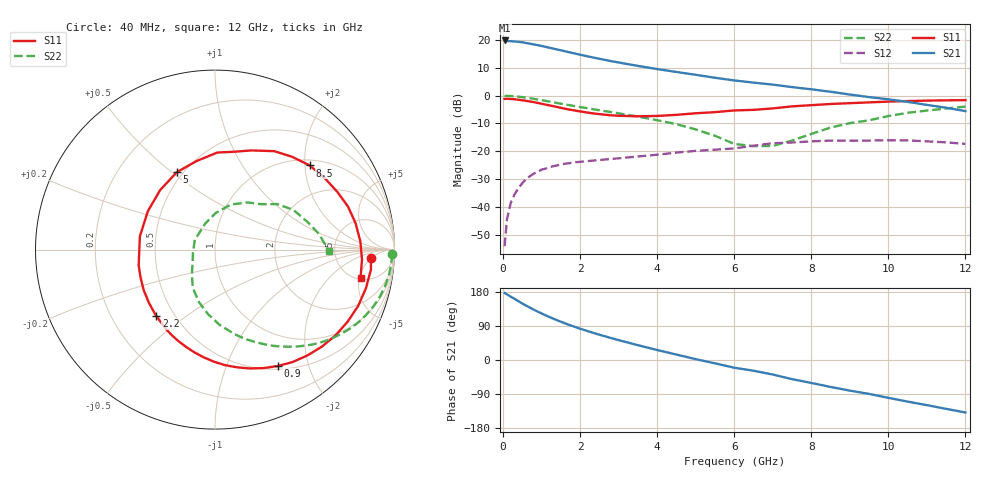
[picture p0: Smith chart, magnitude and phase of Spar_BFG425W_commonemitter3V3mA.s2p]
! Filename: 33bfg425.001
! BFG425W Field C1
! V1=8.136E-001V,V2=3.000E+000V, I1=3.574E-005A, I2=3.000E-003A
# GHz  S  MA  R 50
!  S11  S21  S12  S22
!Freq(GHz)  Mag  Ang  Mag  Ang  Mag  Ang  Mag  Ang
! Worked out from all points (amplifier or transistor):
!   44 points, 40 MHz to 12 GHz, reference 50 ohm
!   highest |S21| = 19.7 dB at 40 MHz (marker M1)
!   |S21| within 3 dB of that: start of sweep to 1.329 GHz
!   unconditionally stable (mu >= 1): 2.826 GHz to end of sweep
!   at 700 MHz: K = 0.24, MSG = 23.7 dB, |S12| = -28.9 dB
!   at 2.4 GHz: K = 0.84, MSG = 18.3 dB, |S12| = -23.2 dB
!   at 12 GHz: K = 1.63, MAG = 1.2 dB, |S12| = -17.3 dB
!   S11 on the Smith chart (normalised r, x): 40 MHz: 12, -5; 900 MHz: 0.54, -1.54; 2.2 GHz: 0.40, -0.39; 5 GHz: 0.46, +0.52; 8.5 GHz: 1.13, +2.12; 12 GHz: 5.23, -5.20
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0.04  0.87 -3.2  9.707 176.7  0.002 71.5  0.986 -1.6
0.1  0.876 -7.2  9.497 173.3  0.006 84.3  0.986 -4.1
0.2  0.868 -14.4  9.419 167.0  0.012 79.6  0.98 -8.2
0.3  0.857 -21.6  9.303 161.3  0.017 75.7  0.969 -12.2
0.5  0.824 -35.5  9.004 149.0  0.027 67.3  0.937 -19.9
0.7  0.783 -48.8  8.485 138.1  0.036 59.6  0.896 -26.9
0.9  0.737 -61.6  8.004 127.7  0.043 52.8  0.849 -33.3
1.2  0.667 -79.5  7.201 113.5  0.052 44.2  0.781 -41.7
1.5  0.603 -96.1  6.461 101.0  0.058 37.2  0.715 -48.9
1.8  0.549 -111.9  5.795 89.6  0.063 31.7  0.657 -55.2
2.2  0.494 -131.5  5.033 76.1  0.067 26.0  0.59 -63.0
2.6  0.457 -150.3  4.414 63.8  0.071 21.8  0.532 -70.3
3  0.434 -168.5  3.908 52.4  0.075 18.2  0.48 -77.4
3.5  0.425 170.0  3.398 39.1  0.081 14.3  0.42 -86.5
4.5  0.451 132.6  2.644 14.3  0.095 5.7  0.307 -106.8
5  0.481 116.2  2.353 2.3  0.102 -0.4  0.247 -120.0
6  0.541 88.6  1.865 -20.3  0.113 -12.3  0.136 -155.9
6.5  0.554 79.5  1.705 -28.3  0.126 -12.0  0.124 -171.9
7.5  0.64 59.0  1.416 -50.5  0.144 -30.3  0.156 109.9
8.5  0.706 41.6  1.17 -71.1  0.156 -46.6  0.267 70.5
10.5  0.797 10.6  0.77 -109.8  0.157 -81.6  0.49 26.8
12  0.826 -11.0  0.526 -138.5  0.136 -112.9  0.633 -0.6
